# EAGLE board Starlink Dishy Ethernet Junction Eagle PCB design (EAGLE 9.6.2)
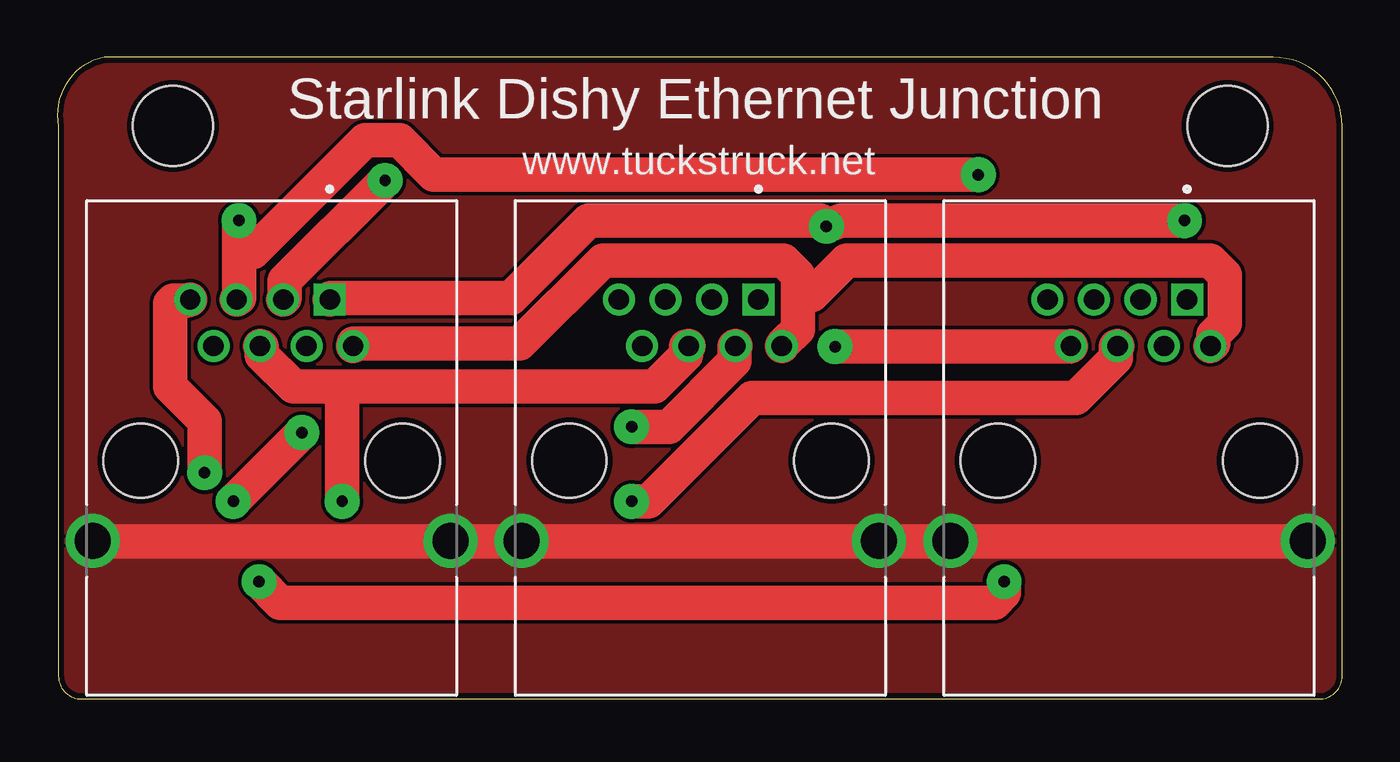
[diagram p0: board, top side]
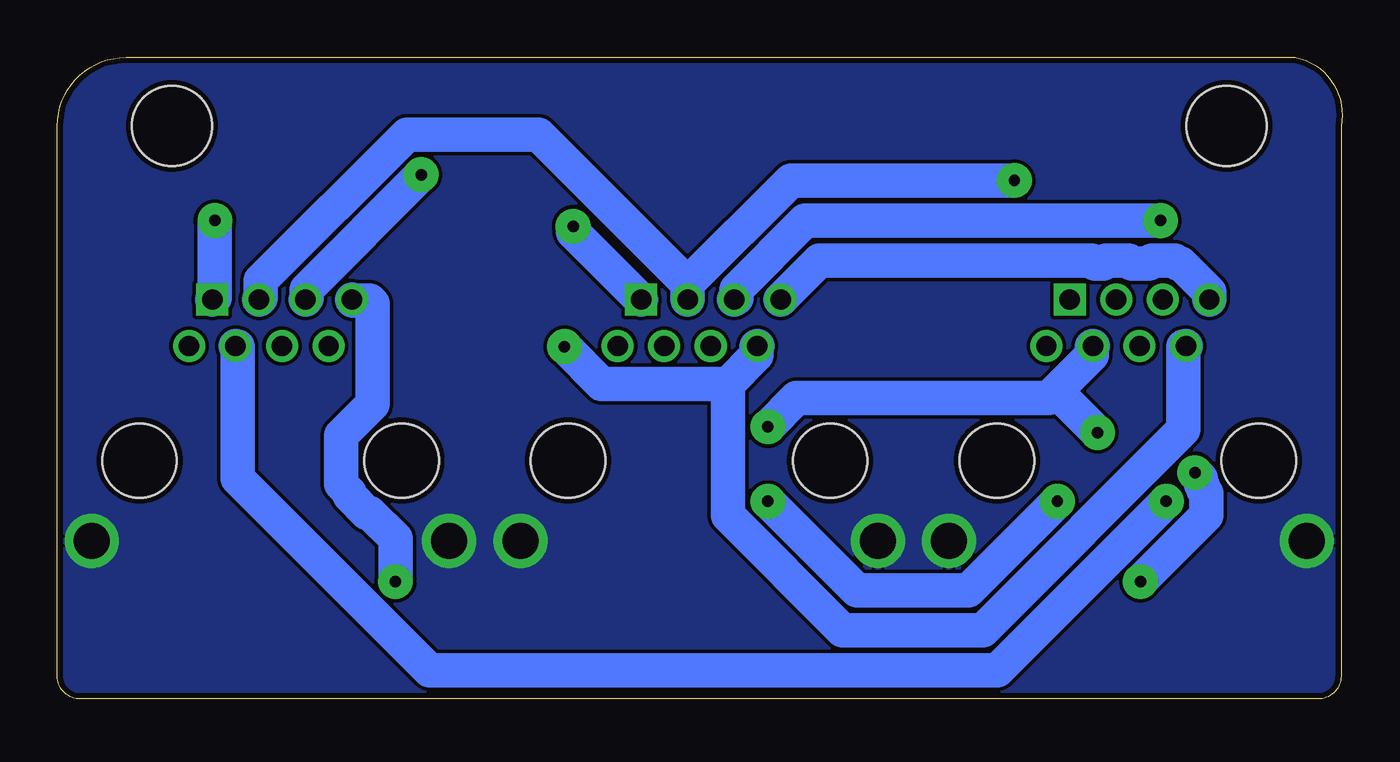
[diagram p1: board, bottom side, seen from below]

Size 56.05 x 28 mm. Coordinates in mm from the lower left corner, seen from the top.
Outline: 0.05,25 0.05,1 arc90 1.05,0 55.05,0 arc90 56.05,1 56.05,25 arc90 53.05,28 2.05,28 arc90 0.05,25
Copper layers (1*16): Top 0.035mm / dielectric 1.63mm / Bottom 0.035mm
Design rules "default *": minimum track width 0.25mm, minimum drill 0.5mm, track to track 0.16mm, track to pad 0.16mm, pad to pad 0.16mm, via to via 0.16mm, smd to smd 0.16mm, copper to edge 0.25mm, drill to drill 0.1322mm, minimum pad ring 10mil, minimum via ring 20mil, stop-mask expansion 4mil, vias tented up to drill 0mil, thermal gap 0mil
Net classes: 0 default: width 1.5 mm
Holes 3.5 mm at 5.05,25 51.05,25

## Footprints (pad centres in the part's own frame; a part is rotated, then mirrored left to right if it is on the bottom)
BEL_SS-60000-009 = drill 0.89 square: 1 2.535,7.03 | drill 0.89: 2 3.555,5; 3 1.525,5; 4 -0.505,5; 5 0.505,7.03; 6 -1.525,7.03; 7 -3.555,7.03; 8 -2.535,5 | drill 1.57: S1 -7.8,-3.51; S2 7.8,-3.51 | hole 3.25: -5.715,0; 5.715,0

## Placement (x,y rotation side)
J1  SS-60000-009  [BEL_SS-60000-009]  46.75,10.4 0 top
J2  SS-60000-009  [BEL_SS-60000-009]  28.05,10.4 0 top
J3  SS-60000-009  [BEL_SS-60000-009]  9.35,10.4 0 top

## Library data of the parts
J1-J3 = SS-60000-009; DESCRIPTION: Jack Modular Connector 8p8c (RJ45, Ethernet) 90° Angle (Right) Shielded Cat6; DIGI-KEY_PART_NUMBER: 380-1096-ND; MF: Stewart Connector; MP: SS-60000-009; PACKAGE: None; PURCHASE-URL: https://pricing.snapeda.com/search/part/SS-60000-009/?ref=eda

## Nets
BI_DA+: J1.1 J2.1 J3.1
BI_DA-: J1.2 J2.2 J3.2
BI_DB+: J1.3 J2.3 J3.3
BI_DB-: J1.6 J2.6 J3.6
BI_DC+: J1.4 J2.4 J3.4
BI_DC-: J1.5 J2.5 J3.5
BI_DD+: J1.7 J2.7 J3.7
BI_DD-: J1.8 J2.8 J3.8
SHIELD: J1.S1 J1.S2 J2.S1 J2.S2 J3.S1 J3.S2

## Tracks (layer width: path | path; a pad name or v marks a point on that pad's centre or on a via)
BI_DA+  (via drill 0.5)
  Top 1.5: J3.1 11.92,17.5 19.8,17.5 23.17,20.88 33.3,20.88 v33.55,20.62 34.17,20.88 v49.17,20.88
  Bottom 1.5: v33.55,20.62 33.55,20.38 30.67,17.5 J2.1 | v49.17,20.88 49.17,17.5 J1.1
BI_DA-
  Top 1.5: 32.3,17.62 32.3,16.12 31.67,15.5 J2.2 | 32.3,17.62 32.3,18.5 31.67,19.12 23.8,19.12 20.17,15.5 12.92,15.5 J3.2 | J1.2 50.42,15.5 50.42,15.88 50.92,16.38 50.92,18.5 50.3,19.12 34.42,19.12 32.92,17.62 32.3,17.62
BI_DB+  (via drill 0.5)
  Top 1.5: v25.05,11.88 26.67,11.88 29.55,14.75 29.55,15.38 J2.3 | v10.67,11.62 v7.67,8.62
  Bottom 1.5: 12.49,13.44 12.8,13.12 23.8,13.12 v25.05,11.88 | 12.49,13.44 10.92,15 10.92,15.38 J3.3 | v7.67,8.62 15.05,1.25 39.8,1.25 48.17,9.62 48.17,15.38 J1.3 | 12.49,13.44 v10.67,11.62
BI_DB-  (via drill 0.5)
  Top 1.5: v7.92,20.88 7.92,19.5 | 7.92,19.5 7.92,17.5 J3.6 | v40.17,22.88 16.42,22.88 14.92,24.38 13.42,24.38 8.55,19.5 7.92,19.5
  Bottom 1.5: v7.92,20.88 23.42,20.88 26.42,17.88 26.42,17.5 J2.6 | v40.17,22.88 45.17,17.88 45.17,17.5 J1.6
BI_DC+  (via drill 0.5)
  Top 1.5: 12.42,13.62 26.05,13.62 27.42,15 27.42,15.38 J2.4 | 12.42,13.62 10.3,13.62 8.92,15 8.92,15.38 J3.4 | v25.05,8.62 25.8,8.62 30.3,13.12 44.42,13.12 46.17,14.88 46.17,15.38 J1.4 | 12.42,13.62 v12.42,8.62
  Bottom 1.5: v25.05,8.62 21.17,4.75 16.3,4.75 v12.42,8.62
BI_DC-  (via drill 0.5)
  Top 1.5: v14.3,22.62 9.92,18.25 9.92,17.5 J3.5
  Bottom 1.5: v14.3,22.62 24.05,22.62 28.55,18.12 | 28.55,18.12 28.55,17.5 J2.5 | 28.55,18.12 35.05,24.62 40.8,24.62 47.17,18.25 47.17,17.5 J1.5
BI_DD+  (via drill 0.5)
  Top 1.5: v41.3,5.12 41.3,4.62 40.87,4.2 9.72,4.2 v8.8,5.12 | v6.42,9.88 6.42,12.12 4.92,13.62 4.92,17.25 5.05,17.38 5.67,17.38 J3.7
  Bottom 1.5: J2.7 22.8,19.12 10.92,19.12 10.8,19 10.42,19 10.3,19.12 9.3,19.12 9.17,19 8.42,19 8.3,19.12 7.3,19.12 7.17,19 7.05,19 5.8,17.75 5.8,17.5 J3.7 | v41.3,5.12 41.3,7 42.42,8.12 42.55,8.12 43.3,8.88 43.3,9 43.67,9.38 43.67,11.5 42.3,12.88 42.3,17.25 42.42,17.38 43.17,17.38 J1.7 | v8.8,5.12 5.92,8 5.92,9 6.05,9.12 6.05,9.25 6.17,9.38 6.17,9.62 v6.42,9.88
BI_DD-  (via drill 0.5)
  Top 1.5: v33.92,15.38 44.17,15.38 J1.8
  Bottom 1.5: 26.8,13.75 26.8,8 21.8,3 15.67,3 6.92,11.75 6.92,15.38 J3.8 | 26.8,13.75 25.55,15 25.55,15.38 J2.8 | v33.92,15.38 32.3,13.75 26.8,13.75
SHIELD
  Top 1.5: J3.S1 1.55,6.88 17.05,6.88 J3.S2 17.8,6.88 20.17,6.88 J2.S1 20.92,6.88 35.17,6.88 J2.S2 35.92,6.88 38.92,6.88 J1.S1 39.67,6.88 54.55,6.88 J1.S2
  pour Top: 57.39,29.05 57.39,-1.46 -1.5,-1.46 -1.5,26.91 0.64,29.05
  pour Bottom: -2.61,29.86 58.77,29.86 58.77,-2.65 -2.61,-2.65

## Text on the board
tNames: Starlink Dishy Ethernet Junction | www.tuckstruck.net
